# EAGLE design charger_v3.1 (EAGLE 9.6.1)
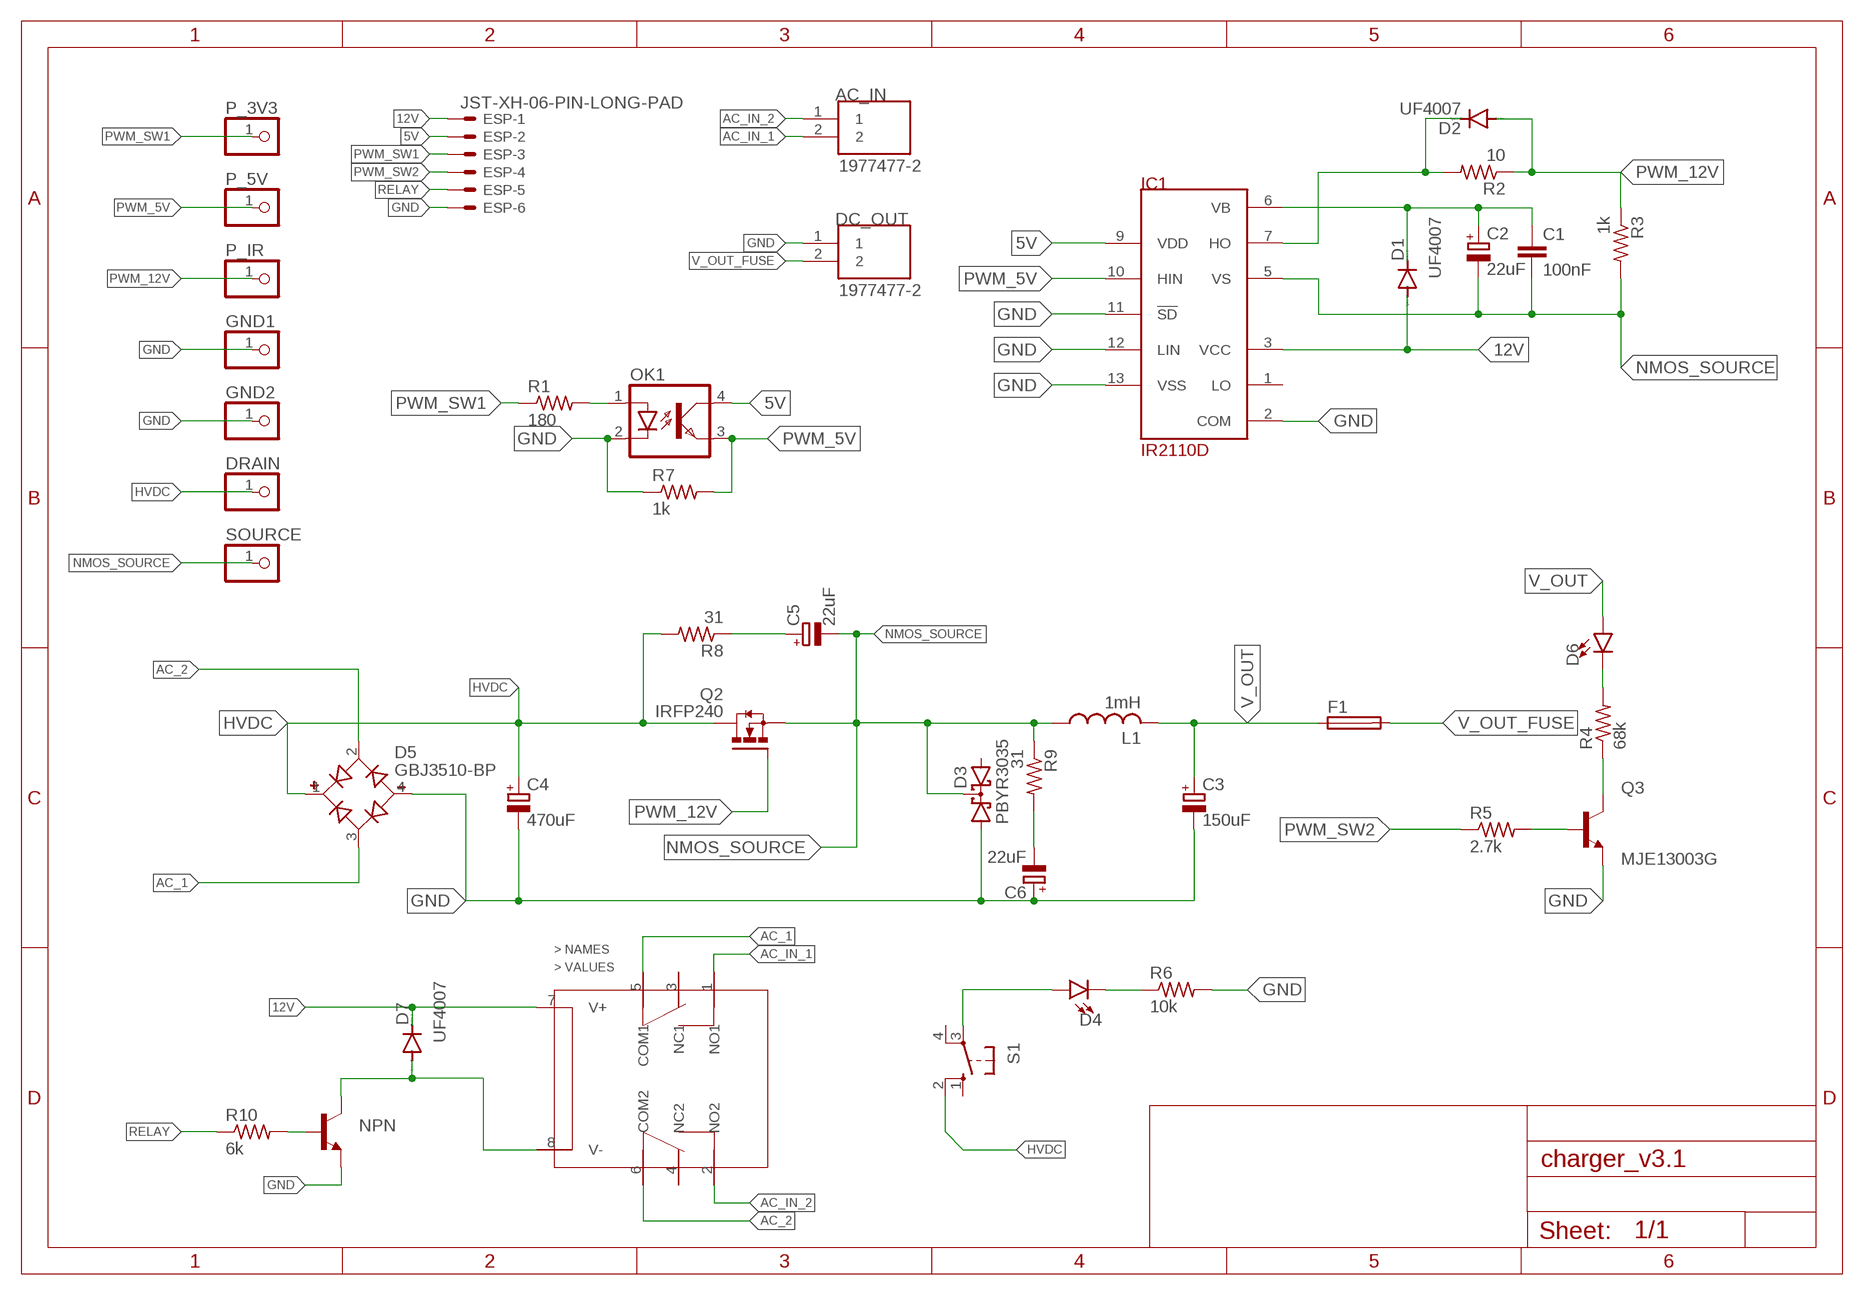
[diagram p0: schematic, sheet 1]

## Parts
AC_IN  1977477-2  [TE_1977477-2]
C1  100nF  C-EU025-025X050  [C025-025X050]
C2  22uF  CPOL-EUE2,5-6E  [E2,5-6E]
C3  150uF  CPOL-EUE7.5-18  [E7,5-18]
C4  470uF  CPOL-EUE10-35  [EB35D]
C5  22uF  CPOL-EUE7.5-18  [E7,5-18]
C6  22uF  CPOL-EUE7.5-18  [E7,5-18]
D1  UF4007  BAS15  [DO34-7]
D2  UF4007  BAS15  [DO34-7]
D3  PBYR3035  [SOT93S]
D4  LED5MM  [LED_5MM]
D5  GBJ3510-BP  [DIOB_GBJ3510-BP]
D6  LED5MM  [LED_5MM]
D7  UF4007  BAS15  [DO34-7]
DC_OUT  1977477-2  [TE_1977477-2]
DRAIN  PINHD-1X1  [1X01]
ESP  JST-XH-06-PIN-LONG-PAD  [JST-XH-06-PACKAGE-LONG-PAD]
F1  FUSEHOLDER  [FUSEHOLDER]
GND1  PINHD-1X1  [1X01]
GND2  PINHD-1X1  [1X01]
IC1  IR2110D  [DIL14]
L1  1mH  L-USTJ7-U1  [TJ7-U1]
NPN  BC547A-NPN-TO92-CBE  [TO92-CBE]
OK1  SFH618A-5  [DIP4]
P_3V3  PINHD-1X1  [1X01]
P_5V  PINHD-1X1  [1X01]
P_IR  PINHD-1X1  [1X01]
Q2  IRFP240  [TO247AC]
Q3  MJE13003G  [TO229P780X300X1364-3]
R1  180  R-US_0204/7  [0204/7]
R2  10  R-US_0204/7  [0204/7]
R3  1k  R-US_0204/7  [0204/7]
R4  68k  R-US_0411/15  [0411/15]
R5  2.7k  R-US_0204/7  [0204/7]
R6  10k  R-US_0204/7  [0204/7]
R7  1k  R-US_0204/7  [0204/7]
R8  31  R-US_0411/15  [0411/15]
R9  31  R-US_0411/15  [0411/15]
R10  6k  R-US_0204/7  [0204/7]
S1  10-XX  [B3F-10XX]
SOURCE  PINHD-1X1  [1X01]
U$1  DPDT-HK19F  [DPDT-HK19F]

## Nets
5V: ESP.2 IC1.9(VDD) OK1.4(COL)
12V: D1.A D7.C ESP.1 IC1.3(VCC) U$1.7(V+)
AC_1: D5.3(AC2) U$1.5(COM1)
AC_2: D5.2(AC1) U$1.6(COM2)
AC_IN_1: AC_IN.2 U$1.1(NO1)
AC_IN_2: AC_IN.1 U$1.2(NO2)
GND: C3.- C4.- C6.+ D3.A1 D5.4(-) DC_OUT.1 ESP.6 GND1.1 GND2.1 IC1.2(COM) IC1.11(!SD) IC1.12(LIN) IC1.13(VSS) NPN.E OK1.2(C) Q3.3(E) R6.2 R7.1
HVDC: C4.+ D5.1(+) DRAIN.1 Q2.2(D) R8.2 S1.2(S1)
N$1: D2.C IC1.7(HO) R2.2
N$2: D4.A S1.3(P)
N$3: Q3.2(C) R4.1
N$4: D6.K(C) R4.2
N$5: Q3.1(B) R5.2
N$6: C5.+ R8.1
N$7: C6.- R9.2
N$8: D4.K(C) R6.1
N$9: OK1.1(A) R1.2
N$13: NPN.B R10.2
N$14: D7.A NPN.C U$1.8(V-)
NMOS_SOURCE: C1.2 C2.- C5.- D3.C IC1.5(VS) L1.1 Q2.3(S) R3.2 R9.1 SOURCE.1
PWM_5V: IC1.10(HIN) OK1.3(EMIT) P_5V.1 R7.2
PWM_12V [pwm_12]: D2.A P_IR.1 Q2.1(G) R2.1 R3.1
PWM_SW1: ESP.3 P_3V3.1 R1.1
PWM_SW2: ESP.4 R5.1
RELAY: ESP.5 R10.1
V_OUT: C3.+ D6.A F1.1 L1.2
V_OUT_FUSE: DC_OUT.2 F1.2
VB: C1.1 C2.+ D1.C IC1.6(VB)
Unconnected: D3.A2 IC1.1(LO) S1.1(S) S1.4(P1) U$1.3(NC1) U$1.4(NC2)

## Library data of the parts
AC_IN DC_OUT = terminal_block_TA:1977477-2: Check availability; AVAILABILITY: In Stock; COMMENT: 1977477-2; DESCRIPTION: Conn Barrier Strip 2 POS 8.25mm Solder ST Thru-Hole 15A/Contact Carton; MF: TE Connectivity; MP: 1977477-2; PACKAGE: None; PRICE: None; PURCHASE-URL: https://pricing.snapeda.com/search/part/1977477-2/?ref=eda
C1 = rcl:C-EU: CAPACITOR, European symbol; SPICEPREFIX: C
C2-C6 = rcl:CPOL-EU: POLARIZED CAPACITOR, European symbol; SPICEPREFIX: C
D1 D2 D7 = diode:BAS15: DIODE
D3 = diode:PBYR3035: Dual DIODE common cathode
D4 D6 = Sparkfun_LED:LED: LED (Generic)
D5 = GBJ3510-BP:GBJ3510-BP: Diode Rectifier Bridge Single 1KV 35A 4-Pin(4+Tab) Case GBJ Bulk/Tube Check availability; AVAILABILITY: In Stock; DESCRIPTION: Bridge Rectifier Single Phase Standard 1 kV Through Hole GBJ; MF: Micro Commercial; MP: GBJ3510-BP; PACKAGE: SIP-4 Micro Commercial Co; PRICE: None; PURCHASE-URL: https://pricing.snapeda.com/search/part/GBJ3510-BP/?ref=eda
DRAIN GND1 GND2 P_3V3 P_5V P_IR SOURCE = pinhead:PINHD-1X1: PIN HEADER
ESP = Rembrandt Electronics - JST XH Connectors v1-0:JST-XH-06-PIN: JST XH Connector 2 Pin Wire to board connector. Pitch: 2,54 mm, (0.100") Number of pins: 6 Created by Rembrandt Electronics www.rembrandtelectronics.com
F1 = TA_library:FUSEHOLDER: FUSE HOLDER; MPN: 0031.7701.11; OC_FARNELL: unknown; OC_NEWARK: 04F1224
IC1 = irs:IR2110
L1 = custom_inductor:L-US: INDUCTOR, American symbol; SPICEPREFIX: L
NPN = transistor:*-NPN-: NPN Transistror BF959 corrected 2008.03.06
OK1 = optocoupler:SFH618?*: Optocoupler, Phototransistor Output, Low Input Current Source: Data sheet; MF: VISHAY/TELEFUNKEN; MPN: SFH618A-5; OC_FARNELL: 1469593; OC_NEWARK: 59K0259
Q2 = IRFP240(TO-247):IRFP240: MOSFET N-CH 200V 20A TO-247AC Check availability; AVAILABILITY: In Stock; DESCRIPTION: N-Channel 200 V 20A (Tc) 150W (Tc) Through Hole TO-247AC; MF: Vishay Siliconix; MP: IRFP240; PACKAGE: TO-247 Vishay Siliconix; PRICE: None
Q3 = MJE13003G:MJE13003G: Bipolar (BJT) Transistor NPN 400V 1.5A 10MHz 1.4W Through Hole TO-225AA Check availability; AVAILABILITY: Not in stock; DESCRIPTION: Bipolar (BJT) Transistor NPN 400 V 1.5 A 10MHz 1.4 W Through Hole TO-126; MF: ON Semiconductor; MP: MJE13003G; PACKAGE: TO-126 ON Semiconductor; PRICE: None
R1-R10 = rcl:R-US_: RESISTOR, American symbol; SPICEPREFIX: R
S1 = switch-omron:10-XX: OMRON SWITCH; MPN: B3F-1000; OC_FARNELL: 176432; OC_NEWARK: 36M3542
U$1 = TA_library:DPDT-HK19F

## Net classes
0 default: width 0.305 mm
1 power: width 6.985 mm, clearance 0.508 mm to class 0
2 pwm_12: width 0.305 mm, clearance 0.508 mm to class 0, clearance 0.508 mm to class 1

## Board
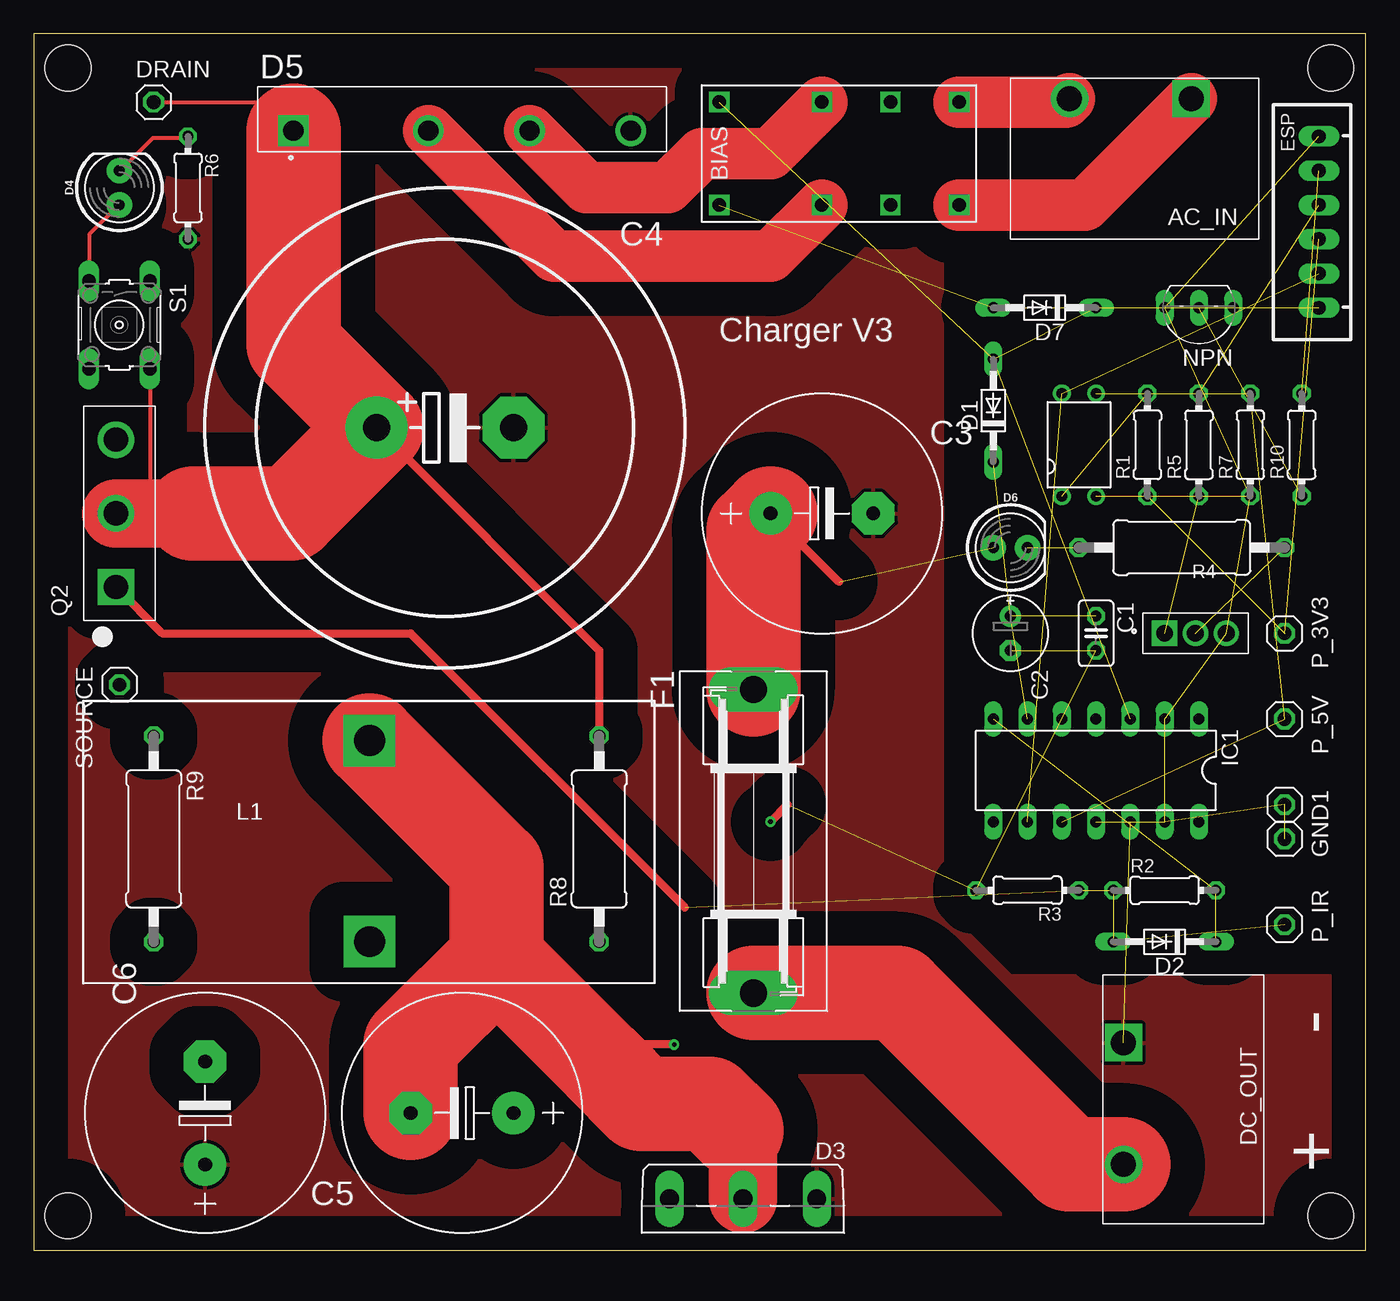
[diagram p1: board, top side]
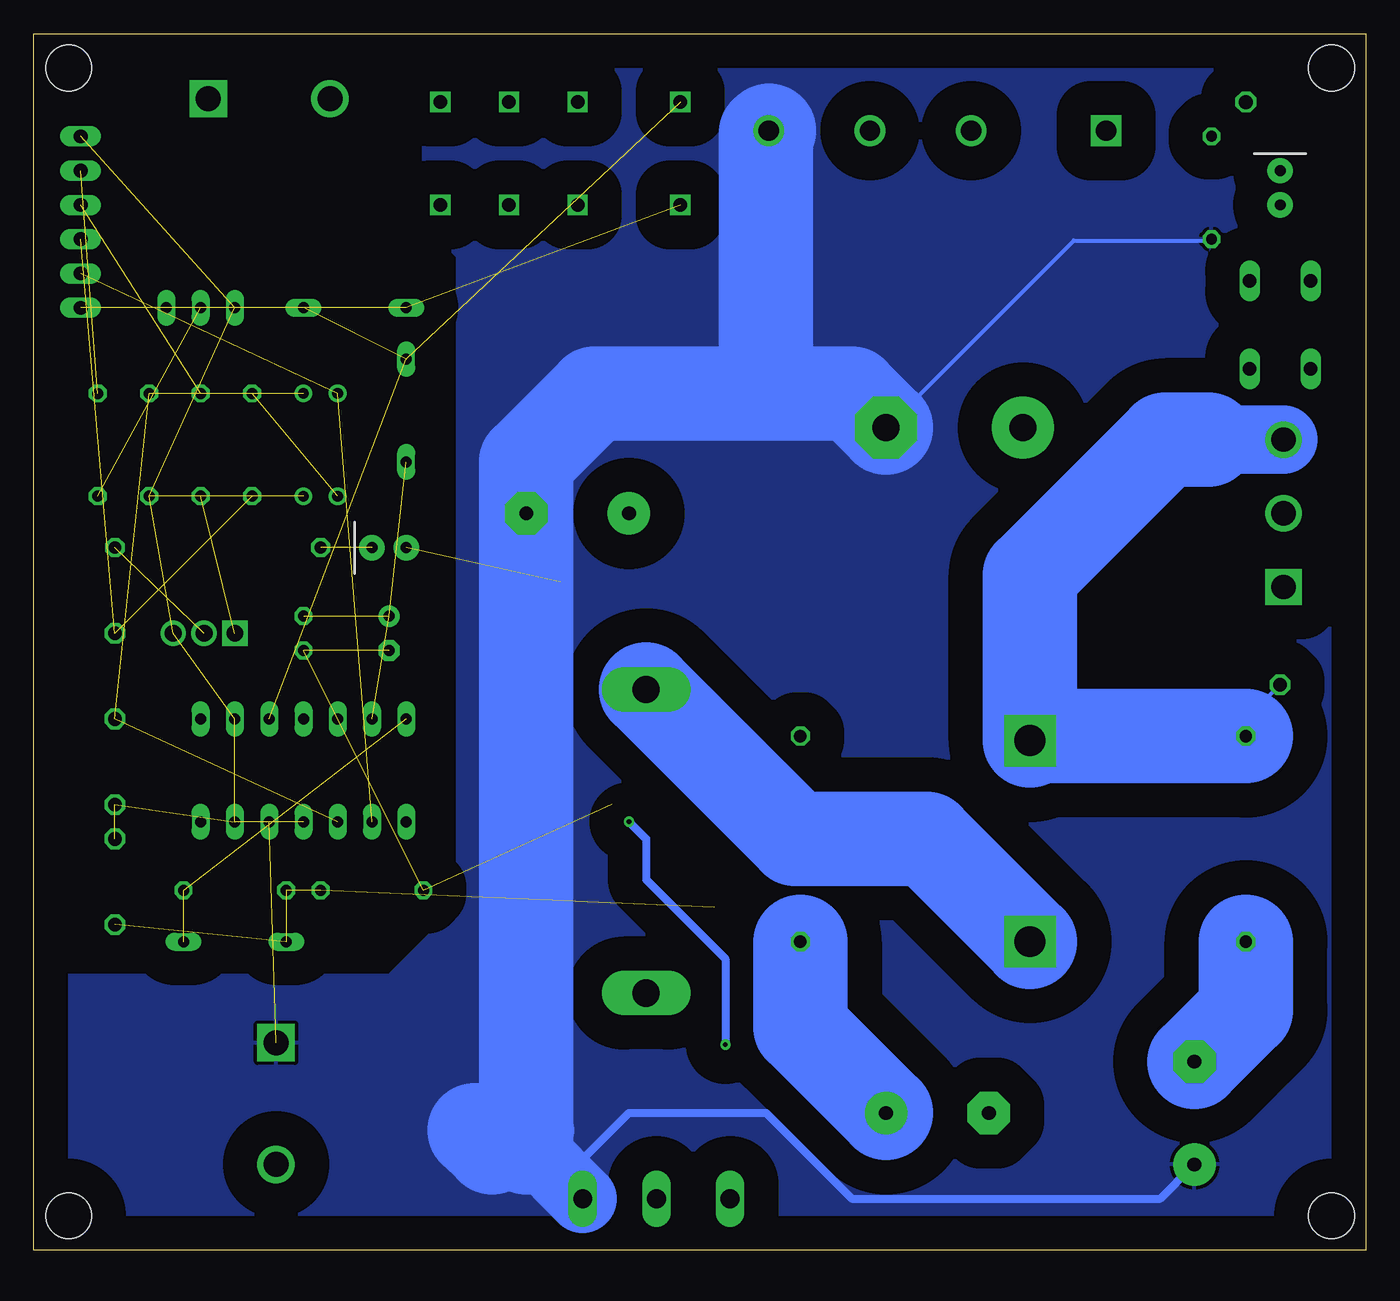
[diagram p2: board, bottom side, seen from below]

Size 98.73 x 90.16 mm. Coordinates in mm from the lower left corner, seen from the top.
Outline: 0,0 98.73,0 98.73,90.16 0,90.16 0,0
Copper layers (1*16): Top 0.035mm / dielectric 1.5mm / Bottom 0.035mm
Design rules "default *": minimum track width 12mil, minimum drill 0.35mm, track to track 12mil, track to pad 12mil, pad to pad 12mil, via to via 12mil, smd to smd 12mil, copper to edge 40mil, drill to drill 6mil, minimum pad ring 10mil, minimum via ring 8mil, stop-mask expansion 4mil, vias tented up to drill 0mil, thermal gap 10mil
Holes 3.4 mm at 2.54,87.63 96.14,87.63 2.54,2.54 96.14,2.54

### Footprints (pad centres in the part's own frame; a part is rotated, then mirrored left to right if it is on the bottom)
TE_1977477-2 = drill 1.85 square: 1 -3.241,-5.334 | drill 1.85: 2 5.781,-5.334
C025-025X050 = drill 0.813 octagon: 1 -1.27,0; 2 1.27,0
E2,5-6E = drill 0.813 pad 1.575: + -1.27,0 | drill 0.813 pad 1.575 octagon: - 1.27,0
E7,5-18 = drill 1.016 pad 3.15: + -3.81,0 | drill 1.016 pad 3.15 octagon: - 3.81,0
EB35D = drill 2.007 pad 4.597: + -5.08,0 | drill 2.007 pad 4.597 octagon: - 5.08,0
DO34-7 = drill 0.813 long: A 3.81,0; C -3.81,0
SOT93S = drill 1.397 long: A1 -5.461,-2.54; A2 5.461,-2.54; C 0,-2.54
LED_5MM = drill 0.813 pad 1.88: A -1.27,0; K 1.27,0
DIOB_GBJ3510-BP = drill 1.51 pad 2.27 square: 1 -12.5,-0.85 | drill 1.51 pad 2.27: 2 -2.5,-0.85; 3 5,-0.85; 4 12.5,-0.85
1X01 = drill 1.016 octagon: 1 0,0
JST-XH-06-PACKAGE-LONG-PAD = drill 1.016 long: 1 -6.35,0; 2 -3.81,0; 3 -1.27,0; 4 1.27,0; 5 3.81,0; 6 6.35,0
FUSEHOLDER = drill 2.007 pad 3.302 long: 1 -11.252,0; 2 11.252,0
DIL14 = drill 0.813 long: 1 -7.62,-3.81; 2 -5.08,-3.81; 3 -2.54,-3.81; 4 0,-3.81; 5 2.54,-3.81; 6 5.08,-3.81; 7 7.62,-3.81; 8 7.62,3.81; 9 5.08,3.81; 10 2.54,3.81; 11 0,3.81; 12 -2.54,3.81; 13 -5.08,3.81; 14 -7.62,3.81
TJ7-U1 = drill 2.286 pad 3.81 square: 1 -6.503,4.826; 2 8.408,4.826
TO92-CBE = drill 0.813 long: B 0,0; C -2.54,0; E 2.54,0
DIP4 = drill 0.8: 1 -1.27,-3.81; 2 1.27,-3.81; 3 1.27,3.81; 4 -1.27,3.81
TO247AC = drill 1.79 pad 2.69 square: 1 -5.46,0.255 | drill 1.79 pad 2.69: 2 0,0.255; 3 5.46,0.255
TO229P780X300X1364-3 = drill 1.25 square: 1 0,0 | drill 1.25: 2 2.29,0; 3 4.58,0
0204/7 = drill 0.813 octagon: 1 -3.81,0; 2 3.81,0
0411/15 = drill 0.914 octagon: 1 -7.62,0; 2 7.62,0
B3F-10XX = drill 1.016 long: 1 -3.251,2.261; 2 3.251,2.261; 3 -3.251,-2.261; 4 3.251,-2.261
DPDT-HK19F = drill 1 square: 1 8.89,3.81; 2 8.89,-3.81; 3 3.81,3.81; 4 3.81,-3.81; 5 -1.27,3.81; 6 -1.27,-3.81; 7 -8.89,3.81; 8 -8.89,-3.81

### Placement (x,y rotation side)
AC_IN  82.55,80.01 180 top
C1  78.74,45.72 270 top
C2  72.39,45.72 270 top
C3  58.42,54.61 0 top
C4  30.48,60.96 0 top
C5  31.75,10.16 180 top
C6  12.7,10.16 90 top
D1  71.12,62.23 90 top
D2  83.82,22.86 180 top
D3  52.58,1.27 180 top
D4  6.35,78.74 90 top
D5  31.75,83.82 0 top
D6  72.39,52.07 0 top
D7  74.93,69.85 180 top
DC_OUT  86.11,12.13 270 top
DRAIN  8.89,85.09 0 top
ESP  95.25,76.2 90 top
F1  53.34,30.3 270 top
GND1  92.71,30.48 0 top
GND2  92.71,33.02 0 top
IC1  78.74,35.56 180 top
L1  20.07,31.27 270 top
NPN  86.36,69.85 180 top
OK1  77.47,59.69 0 top
P_3V3  92.71,45.72 90 top
P_5V  92.71,39.37 90 top
P_IR  92.71,24.13 90 top
Q2  6.35,54.61 90 top
Q3  83.82,45.72 0 top
R1  82.55,59.69 90 top
R2  83.82,26.67 0 top
R3  73.66,26.67 180 top
R4  85.09,52.07 180 top
R5  86.36,59.69 270 top
R6  11.43,78.74 270 top
R7  90.17,59.69 90 top
R8  41.91,30.48 90 top
R9  8.89,30.48 270 top
R10  93.98,59.69 270 top
S1  6.35,68.58 270 top
SOURCE  6.35,41.91 0 top
U$1  59.69,81.28 0 top

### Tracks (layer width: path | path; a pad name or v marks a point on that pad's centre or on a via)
5V  (2 unrouted)
12V  (4 unrouted)
AC_1
  Top 3.81: D5.3 40.98,78.74 46.99,78.74 49.53,81.28 54.61,81.28 U$1.5
AC_2
  Top 3.81: U$1.6 54.61,73.66 38.56,73.66 D5.2
AC_IN_1
  Top 3.81: U$1.1 76.52,85.09 AC_IN.2
AC_IN_2
  Top 3.81: U$1.2 77.92,77.47 AC_IN.1
GND  (11 unrouted)
  Top 0.305: 35.66,60.96 C4.-
  Bottom 0.305: R6.2 11.43,74.83 21.64,74.83 35.51,60.96 C4.- | 44.2,82.91 D5.4 46.85,80.37 | D3.A1 58.04,6.25 | 12.8,6.25 C6.+
  Bottom 0.61: D3.A1 58.04,6.73 54.61,10.16 44.45,10.16 38.1,3.81 15.24,3.81 12.8,6.25
  Bottom 3.81: 60.58,8.89 66.04,8.89
  Bottom 5.08: D3.A1 61.85,7.62 62.23,7.62 64.77,7.62
  Bottom 6.985: 64.77,7.62 66.04,8.89 | C4.- 38.1,63.5 44.45,63.5 | D5.4 44.45,82.77 44.45,63.5 | 44.45,63.5 57.15,63.5 62.23,58.42 C3.- 62.23,7.62
  pour Top (isolate 2.54): -10.16,95.25 69.85,95.25 69.85,76.2 67.31,73.66 67.31,25.4 72.39,20.32 97.79,20.32 99.06,19.05 99.06,-7.62 -10.16,-7.62
  pour Bottom (isolate 2.54): -12.7,97.79 69.85,97.79 69.85,76.2 67.31,73.66 67.31,25.4 72.39,20.32 97.79,20.32 99.06,19.05 99.06,-7.62 -12.7,-7.62
HVDC
  Top 0.305: 8.69,54.61 8.69,56.99 | 8.69,56.99 8.69,65.23 S1.2 | 8.69,56.99 8.73,56.99 8.73,54.61 | DRAIN.1 17.13,85.09 D5.1
  Top 0.61: R8.2 41.91,44.45 C4.+
  Top 5.08: Q2.2 8.73,54.61 11.81,54.61
  Top 6.985: D5.1 19.25,67.11 C4.+ 19.05,54.61 11.81,54.61
N$1  (2 unrouted)
N$2
  Top 0.305: S1.3 4.12,71.93 4.12,75.29 6.25,77.42 D4.A
N$3  (1 unrouted)
N$4  (1 unrouted)
N$5  (1 unrouted)
N$6
  Bottom 6.985: R8.1 41.91,16.51 C5.+
N$7
  Bottom 6.985: C6.- 8.89,17.78 R9.2
N$8
  Top 0.305: R6.1 11.43,82.45 8.84,82.45 6.4,80.01 D4.K
N$9  (1 unrouted)
N$13  (1 unrouted)
N$14  (2 unrouted)
NMOS_SOURCE  (via drill 0.35)  (4 unrouted)
  Top 0.61: 55.88,33.02 v54.61,31.75 | v47.47,15.24 43.66,15.24 42.15,13.73
  Top 5.08: D3.C 52.58,8.38 52.07,8.89
  Top 6.985: L1.1 34.29,28.37 34.29,21.59 | 34.29,21.59 42.15,13.73 45.02,10.86 50.1,10.86 52.07,8.89 | C5.- 27.94,15.24 34.29,21.59
  Bottom 0.305: SOURCE.1 8.89,39.37 R9.1
  Bottom 0.61: v47.47,15.24 47.47,21.59 53.34,27.46 53.34,30.48 v54.61,31.75
  Bottom 5.08: Q2.3 11.68,60.07
  Bottom 6.985: 11.68,60.07 14.86,60.07 24.89,50.04 L1.1 24.56,38.1 R9.1
PWM_5V  (3 unrouted)
PWM_12V  (4 unrouted)
  Top 0.61: Q2.1 9.53,45.72 27.94,45.72 48.26,25.4
PWM_SW1  (2 unrouted)
PWM_SW2  (1 unrouted)
RELAY  (1 unrouted)
V_OUT  (1 unrouted)
  Top 0.61: 59.69,49.53 C3.+
  Top 6.985: C3.+ 53.34,53.34 F1.1
  Bottom 6.985: L1.2 32.51,30.48 42.27,30.48 F1.1
V_OUT_FUSE
  Top 6.985: F1.2 64.01,19.05 76.71,6.35 DC_OUT.2
VB  (3 unrouted)

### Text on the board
tPlace: - | +
tNames: Charger V3

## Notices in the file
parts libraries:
Sparkfun_LED: Licensing: Creative Commons ShareAlike 4.0 International - https://creativecommons.org/licenses/by-sa/4.0
